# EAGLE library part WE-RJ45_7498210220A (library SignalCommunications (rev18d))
WE-RJ45 LAN Transformer Order Code 7498210220A Design SMD xBase-T 10/100 Base-T Ports 1x1 Application Standard Tab Position Vertical LED (Left-Right) GREEN-GREEN EMI Fingers No Details see: http://katalog.we-online.de/en/pbs/WE-LAN-RJ45 Created by Yingchun Shan 2016 (C) Wurth Elektronik
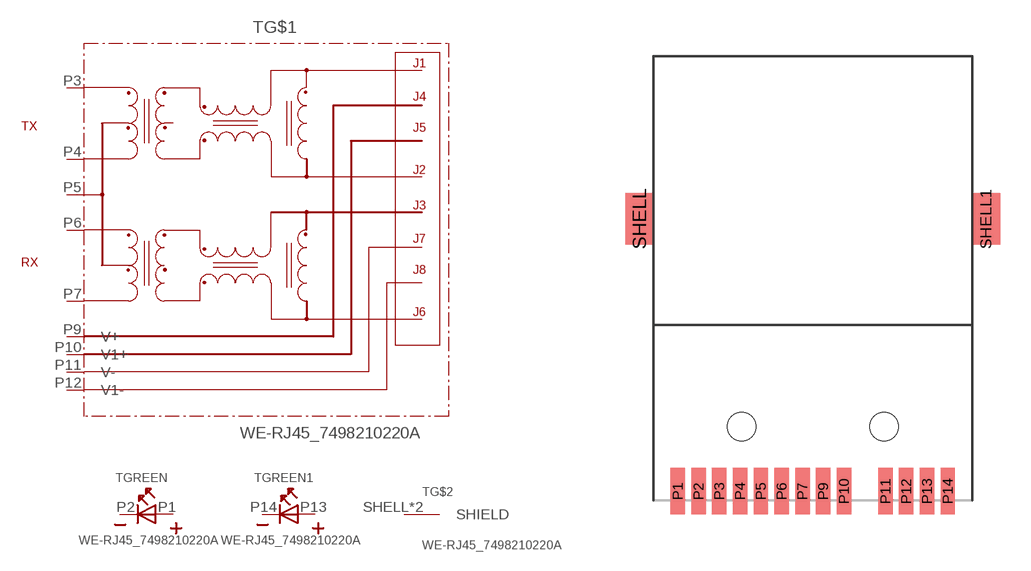
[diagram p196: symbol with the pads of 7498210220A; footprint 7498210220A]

Designator prefix T; gates G$1=7498210220A GREEN=LED_2PIN GREEN1=LED_2PIN G$2=SHIELD

## WE-RJ45_7498210220A  [7498210220A]
P1  GREEN:A  pas
P2  GREEN:K  pas
P3  G$1:P3
P4  G$1:P4
P5  G$1:P5
P6  G$1:P6
P7  G$1:P7
P9  G$1:V+
P10  G$1:V1+
P11  G$1:V-
P12  G$1:V1-
P13  GREEN1:A  pas
P14  GREEN1:K  pas
SHELL  G$2:SHIELD  pas
SHELL1  G$2:SHIELD  pas

## Footprint 7498210220A (pad centres in mm)
smd 0.71 x 2.29: P1 -6.63,-3.18; P2 -5.61,-3.18; P3 -4.59,-3.18; P4 -3.57,-3.18; P5 -2.55,-3.18; P6 -1.53,-3.18; P7 -0.51,-3.18; P9 0.51,-3.18; P10 1.53,-3.18; P11 3.57,-3.18; P12 4.59,-3.18; P13 5.61,-3.18; P14 6.63,-3.18
smd 1.4 x 2.54: SHELL -8.51,10.2; SHELL1 8.51,10.2
hole 1.4 at -3.5,0
hole 1.4 at 3.5,0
